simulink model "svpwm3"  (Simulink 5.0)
settings: Solver=ode45  StartTime=0  StopTime=.02  MaxStep=1e-6  RelTol=1e-3
InitFcn:
  | warning off;clc;fout=50;fsw=20000;disp(' Output frequency Switching frequency  [Hz] :  ');
  | disp('         fout       fsw');disp([fout   fsw])
libraries: simulink x3, simulink_extras x1

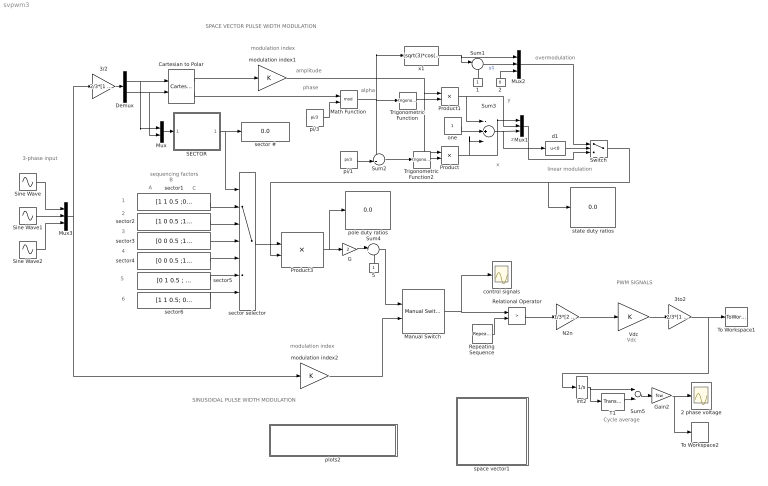
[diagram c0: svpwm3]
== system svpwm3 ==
  note: SPACE VECTOR PULSE WIDTH MODULATION
  note: amplitude
  note: phase
  note: sequencing factors
  note: 1
  note: 2
  note: 3
  note: 4
  note: 5
  note: 6
  note: A
  note: B
  note: C
  note: alpha
  note: y
  note: x
  note: modulation index
  note: PWM SIGNALS
  note: z
  note: overmodulation
  note: linear modulation
  note: Cycle average
  note: SINUSOIDAL PULSE WIDTH MODULATION
  note: modulation index
  note: 3-phase input
  note: Vdc
  1 : Constant  Orientation=up
  2 : Constant  Orientation=up  Value=0
  2 phase voltage : Scope
  3/2 : Gain  Gain=2/3*[1 -0.5 -0.5;0 sqrt(3)/2 -sqrt(3)/2]  Multiplication=Matrix(K*u)
  3to2 : Gain  Gain=2/3*[1 -0.5 -0.5;0 sqrt(3)/2 -sqrt(3)/2]  Multiplication=Matrix(K*u)
  5 : Constant  Orientation=up
  Cartesian to Polar : simulink_extras/Transformations/Cartesian to Polar
  Demux : Demux  Outputs=2
  G : Gain  Gain=2
  Gain2 : Gain  Gain=fsw
  Manual Switch : simulink/Signal Routing/Manual Switch  sw=1  action=0
  Math Function : Math  Operator=mod
  Mux : Mux  Inputs=2
  Mux1 : Mux  Inputs=3
  Mux2 : Mux  Inputs=3
  Mux3 : Mux  Inputs=3
  N2n : Gain  Gain=1/3*[2 -1 -1;-1 2 -1;-1 -1 2]  Multiplication=Matrix(K*u)
  Product : Product
  Product1 : Product
  Product3 : Product  Multiplication=Matrix(*)
  Relational Operator : RelationalOperator  Operator=>
  Repeating Sequence : simulink/Sources/Repeating Sequence  rep_seq_t="[0  0.5/fsw 1/fsw]"  rep_seq_y=[1 -1 1]
  SECTOR : Subsystem
  Sine Wave : Sin  Frequency=2*pi*fout  Phase=pi/2  SampleTime=0
  Sine Wave1 : Sin  Frequency=2*pi*fout  Phase=pi/2 -2*pi/3  SampleTime=0
  Sine Wave2 : Sin  Frequency=2*pi*fout  Phase=pi/2+2*pi/3  SampleTime=0
  Sum1 : Sum  Inputs=|-+
  Sum2 : Sum  Inputs=-+|
  Sum3 : Sum  Inputs=-+-|
  Sum4 : Sum  Inputs=|+-
  Sum5 : Sum  Inputs=+-
  Switch : Switch  Threshold=0.5
  T1 : TransportDelay  DelayTime=1/fsw
  To Workspace1 : ToWorkspace  VariableName=abpwm  SampleTime=-1  SaveFormat=Array
  To Workspace2 : ToWorkspace  VariableName=ab  SampleTime=-1  SaveFormat=Array
  Trigonometric Function : Trigonometry
  Trigonometric Function2 : Trigonometry
  Vdc : Gain
  control signals : Scope
  d1 : Fcn  Expr=u<0
  int2 : Integrator
  modulation index1 : Gain
  modulation index2 : Gain
  one : Constant
  pi/1 : Constant  Value=pi/3
  pi/3 : Constant  Value=pi/3
  plots2 : Subsystem
  pole duty ratios : Display
  sector selector : MultiPortSwitch  Inputs=6
  sector # : Display
  sector1 : Constant  Value=[1 1 0.5 ;0 1 0.5;0 0 0.5]
  sector2 : Constant  Value=[1 0 0.5 ;1 1 0.5; 0 0 0.5]  VectorParams1D=off
  sector3 : Constant  Value=[0 0 0.5 ;1 1 0.5; 0 1 0.5]  VectorParams1D=off
  sector4 : Constant  Value=[0 0 0.5 ;1 0 0.5; 1 1 0.5]
  sector5 : Constant  Value=[0 1 0.5 ; 0 0 0.5; 1 1 0.5]  VectorParams1D=off
  sector6 : Constant  Value=[1 1 0.5; 0 0 0.5; 1 0 0.5]  VectorParams1D=off
  space vector1 : Subsystem
  state duty ratios : Display
  x1 : Fcn  Expr=(sqrt(3)*cos(u)-sin(u))/(sqrt(3)*cos(u)+sin(u))
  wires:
  sector2/1 -> sector selector/3
  sector1/1 -> sector selector/2
  sector3/1 -> sector selector/4
  5/1 -> Sum4/2
  G/1 -> Sum4/1
  pi/1/1 -> Sum2/2
  Math Function/1 -> Trigonometric Function/1, Sum2/1, x1/1
  Sum2/1 -> Trigonometric Function2/1
  Trigonometric Function/1 -> Product1/2
  Trigonometric Function2/1 -> Product/2
  modulation index1/1 -> Product/1, Product1/1
  Demux/2 -> Cartesian to Polar/2, Mux/2
  Demux/1 -> Cartesian to Polar/1, Mux/1
  pi/3/1 -> Math Function/2
  Cartesian to Polar/1 -> modulation index1/1
  Product1/1 -> Mux1/2, Sum3/1
  Product/1 -> Mux1/1, Sum3/3
  Cartesian to Polar/2 -> Math Function/1
  sector4/1 -> sector selector/5
  sector5/1 -> sector selector/6
  sector6/1 -> sector selector/7
  one/1 -> Sum3/2
  Sum3/1 -> Mux1/3, d1/1
  Mux/1 -> SECTOR/1(vab)
  SECTOR/1(sector) -> sector selector/1, sector #/1
  sector selector/1 -> Product3/1
  Product3/1 -> G/1, pole duty ratios/1
  d1/1 -> Switch/2
  x1/1 -> Mux2/1, Sum1/1
  Sum1/1 -> Mux2/2  "y1"
  2/1 -> Mux2/3
  1/1 -> Sum1/2
  Mux1/1 -> Switch/3
  Mux2/1 -> Switch/1
  Switch/1 -> Product3/2, state duty ratios/1
  Repeating Sequence/1 -> Relational Operator/2
  T1/1 -> Sum5/2
  int2/1 -> Sum5/1, T1/1
  Sum5/1 -> Gain2/1
  Gain2/1 -> 2 phase voltage/1, To Workspace2/1
  Sine Wave/1 -> Mux3/1
  Sine Wave1/1 -> Mux3/2
  Sine Wave2/1 -> Mux3/3
  Sum4/1 -> Manual Switch/1
  Manual Switch/1 -> Relational Operator/1, control signals/1
  modulation index2/1 -> Manual Switch/2
  Mux3/1 -> modulation index2/1, 3/2/1
  3/2/1 -> Demux/1
  3to2/1 -> To Workspace1/1, int2/1
  Vdc/1 -> 3to2/1
  Relational Operator/1 -> N2n/1
  N2n/1 -> Vdc/1

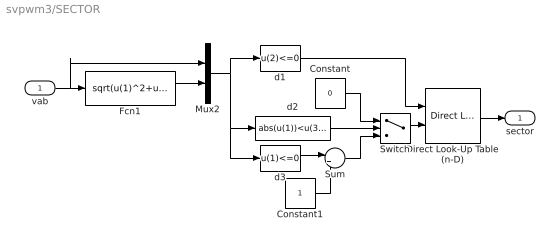
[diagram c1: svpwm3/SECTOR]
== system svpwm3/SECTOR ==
  vab : Inport
  Constant : Constant  Value=0
  Constant1 : Constant
  Direct Look-Up Table (n-D) : simulink/Look-Up Tables/Direct Look-Up Table (n-D)  maskTabDims=2  explicitNumDims=1  outDims=Element  tabIsInput=off  mxTable=[2 1 3;5 6 4]  clipFlag=Warning
  Fcn1 : Fcn  Expr=sqrt(u(1)^2+u(2)^2)
  Mux2 : Mux  Inputs=2
  Sum : Sum  Inputs=|++
  Switch : Switch  Threshold=0.5
  d1 : Fcn  Expr=u(2)<=0
  d2 : Fcn  Expr=abs(u(1))<u(3)/2
  d3 : Fcn  Expr=u(1)<=0
  sector : Outport
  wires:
  Fcn1/1 -> Mux2/2
  d2/1 -> Switch/2
  Switch/1 -> Direct Look-Up Table (n-D)/2
  d1/1 -> Direct Look-Up Table (n-D)/1
  d3/1 -> Sum/1
  Constant1/1 -> Sum/2
  Sum/1 -> Switch/3
  Constant/1 -> Switch/1
  vab/1 -> Fcn1/1, Mux2/1
  Direct Look-Up Table (n-D)/1 -> sector/1
  Mux2/1 -> d1/1, d2/1, d3/1

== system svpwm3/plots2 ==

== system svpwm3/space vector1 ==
